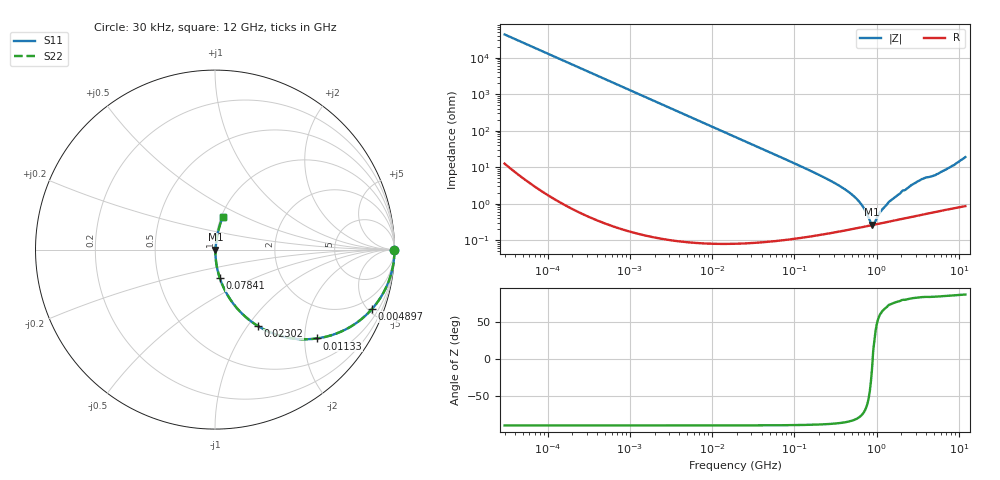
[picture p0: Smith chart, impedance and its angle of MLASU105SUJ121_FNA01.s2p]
! MLASU105SUJ121_FNA01  S-PARAMETER MODEL  ( General Type )
! Model Generated by TAIYO YUDEN Corporation (http://www.ty-top.com)
! Version 3.0
! TAIYO YUDEN Control No. 120810
! Copyright(c) 2003 TAIYO YUDEN CO.,LTD. All Rights Reserved.
! Product Description (link to TY-COMPAS)
! https://ds.yuden.co.jp/TYCOMPAS/or/detail?pn=MLASU105SUJ121JFNA01&u=M
! Products Name : Multilayer Ceramic Capacitors
! Characteristics :
!  Capacitance : 120 pF , Rated Voltage : 50V , TCC : UJ / U2J
!  Case Size : 1.0 x 0.5 / 0.039 x 0.02 [mm/inch] , Thickness : 0.5 / 0.02 [mm/inch]
!  (Conditions: Temperature = 25 degC , DC Bias Current/Voltage = 0A / 0V)
! External Node Assignments :
!  1  o---| |---o  2
! GND o---------o GND
! Frequency Range : 0.03MHz  -  12000MHz  [ 401 STEP ]
# MHz S RI R 50
! Freq[MHz].  S11 Real  S11 Imag  S21 Real  S21 Imag  S12 Real  S12 Imag  S22 Real  S22 Imag
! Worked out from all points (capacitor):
!   401 points, 30 kHz to 12 GHz, reference 50 ohm
!   read as one part in series: C = 123 pF near 32 kHz
!   lowest |Z| = 266 mohm at 880.6 MHz (marker M1)
!   series resonance near 895.2 MHz, so ESL is about 260 pH
!   S11 on the Smith chart (normalised r, x): 30 kHz: open; 4.897 MHz: 1.00, -5.29; 11.33 MHz: 1.00, -2.29; 23.02 MHz: 1.00, -1.12; 78.41 MHz: 1.00, -0.33; 12 GHz: 1.02, +0.38
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0.03  1 -0.00232  6.04e-06 0.00232  6.04e-06 0.00232  1 -0.00232
0.260295  0.9996 -0.0201  0.000406 0.0201  0.000406 0.0201  0.9996 -0.0201
0.915519  0.995 -0.0704  0.00499 0.0704  0.00499 0.0704  0.995 -0.0704
2.258455  0.9704 -0.1693  0.0296 0.1693  0.0296 0.1693  0.9704 -0.1693
4.897055  0.8747 -0.3309  0.1253 0.3309  0.1253 0.3309  0.8747 -0.3309
7.447352  0.7512 -0.4321  0.2488 0.4321  0.2488 0.4321  0.7512 -0.4321
11.3258  0.5663 -0.4952  0.4337 0.4952  0.4337 0.4952  0.5663 -0.4952
18.97367  0.3176 -0.465  0.6824 0.465  0.6824 0.465  0.3176 -0.465
23.02407  0.2402 -0.4265  0.7598 0.4265  0.7598 0.4265  0.2402 -0.4265
39.83545  0.0958 -0.293  0.9042 0.293  0.9042 0.293  0.0958 -0.293
78.41115  0.0271 -0.1592  0.9729 0.1592  0.9729 0.1592  0.0271 -0.1592
164.6252  0.00701 -0.0754  0.993 0.0754  0.993 0.0754  0.00701 -0.0754
324.0443  0.00287 -0.0346  0.9971 0.0346  0.9971 0.0346  0.00287 -0.0346
508.9517  0.00232 -0.0172  0.9977 0.0172  0.9977 0.0172  0.00232 -0.0172
658.7456  0.00235 -0.00903  0.9976 0.00903  0.9976 0.00903  0.00235 -0.00903
880.5704  0.00259 -0.000564  0.9974 0.000564  0.9974 0.000564  0.00259 -0.000564
939.2353  0.00267 0.0012  0.9973 -0.0012  0.9973 -0.0012  0.00267 0.0012
1139.739  0.00295 0.00568  0.997 -0.00568  0.997 -0.00568  0.00295 0.00568
1428.372  0.00337 0.0111  0.9966 -0.0111  0.9966 -0.0111  0.00337 0.0111
2998.885  0.00601 0.0373  0.994 -0.0373  0.994 -0.0373  0.00601 0.0373
5534.236  0.0103 0.0647  0.9897 -0.0647  0.9897 -0.0647  0.0103 0.0647
12000  0.0425 0.1804  0.9575 -0.1804  0.9575 -0.1804  0.0425 0.1804
